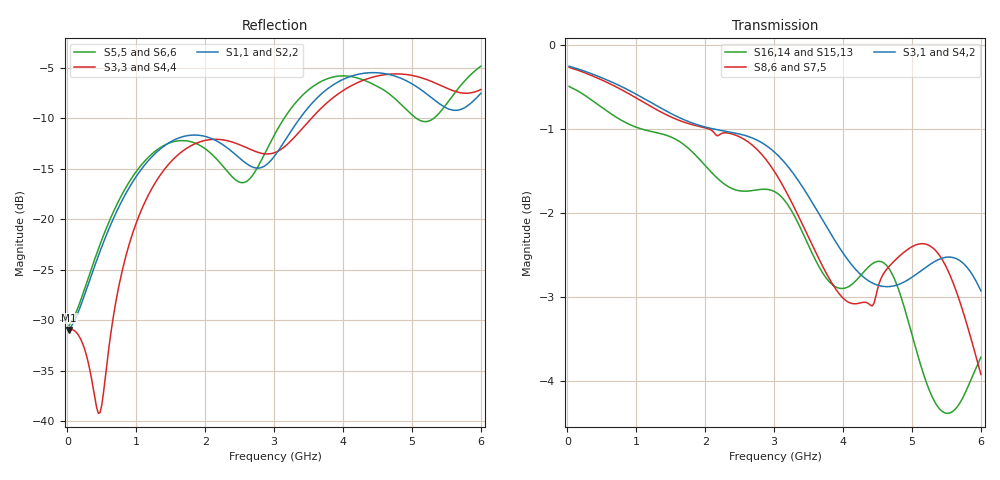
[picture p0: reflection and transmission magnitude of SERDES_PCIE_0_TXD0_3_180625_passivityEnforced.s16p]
! RTG4 CQ352 S-parameter file
! Microsemi Corporation (c) 2019
!Initial ver: Feb 12, 2019
! Port::NET_NAME::S-parameter ports::PORT SIDE
! Port1::SERDES_PCIE_0_TXD0_N::1::DIE
! Port2::SERDES_PCIE_0_TXD0_P::2::DIE
! Port3::SERDES_PCIE_0_TXD0_N::3::Lead
! Port4::SERDES_PCIE_0_TXD0_P::4::Lead
! Port5::SERDES_PCIE_0_TXD1_N::5::DIE
! Port6::SERDES_PCIE_0_TXD1_P::6::DIE
! Port7::SERDES_PCIE_0_TXD1_N::7::Lead
! Port8::SERDES_PCIE_0_TXD1_P::8::Lead
! Port9::SERDES_PCIE_0_TXD2_N::9::DIE
! Port10::SERDES_PCIE_0_TXD2_P::10::DIE
! Port11::SERDES_PCIE_0_TXD2_N::11::Lead
! Port12::SERDES_PCIE_0_TXD2_P::12::Lead
! Port13::SERDES_PCIE_0_TXD3_N::13::DIE
! Port14::SERDES_PCIE_0_TXD3_P::14::DIE
! Port15::SERDES_PCIE_0_TXD3_N::15::Lead
! Port16::SERDES_PCIE_0_TXD3_P::16::Lead
!PowerSI Version: 17.0.2.03131.86335  002
!Computer Host Name: W764D-PINDIS
!TouchstoneFormatFlag = 1
! GNDNET
! NETSLIST
!User Comments:
!  Touchstone file from project YBDH07-1_op7_160920_TXD_0-3
!  Exported from HFSS 2016.2.0
!  Terminal data exported
!  Port[1] = FC_SERDES_PCIE_0_TXD0_N_T1
!  Port[2] = FC_SERDES_PCIE_0_TXD0_P_T1
!  Port[3] = LEAD_9_36_T1
!  Port[4] = LEAD_9_35_T1
!  Port[5] = FC_SERDES_PCIE_0_TXD1_N_T1
!  Port[6] = FC_SERDES_PCIE_0_TXD1_P_T1
!  Port[7] = LEAD_9_28_T1
!  Port[8] = LEAD_9_27_T1
!  Port[9] = FC_SERDES_PCIE_0_TXD2_N_T1
!  Port[10] = FC_SERDES_PCIE_0_TXD2_P_T1
!  Port[11] = LEAD_9_T1
!  Port[12] = LEAD_T1
!  Port[13] = FC_SERDES_PCIE_0_TXD3_N_T1
!  Port[14] = FC_SERDES_PCIE_0_TXD3_P_T1
!  Port[15] = LEAD_4_T1
!  Port[16] = LEAD_6_T1
#	Hz	S	DB	R	50
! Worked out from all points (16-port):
!   240 points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, 25 MHz to 6 GHz, reference 50 ohm
!   strongest paths, dB at 25 MHz, 1.525 GHz, 3.025 GHz, 4.525 GHz, 6 GHz:
!     S3,1: -0.2, -0.8, -1.3, -2.9, -2.9
!     S4,2: -0.2, -0.8, -1.3, -2.9, -2.9
!     S8,6: -0.3, -0.9, -1.5, -2.8, -3.9
!     S7,5: -0.3, -0.9, -1.5, -2.7, -4.0
!     S16,14: -0.5, -1.1, -1.8, -2.6, -3.7
!     S15,13: -0.5, -1.1, -1.8, -2.6, -3.8
!   lowest |S11| = -31.0 dB at 25 MHz (marker M1), VSWR 1.06, Z = 52.9 + j0.0358 ohm
!   |S11| at or under -10 dB: start of sweep to 3.375 GHz
